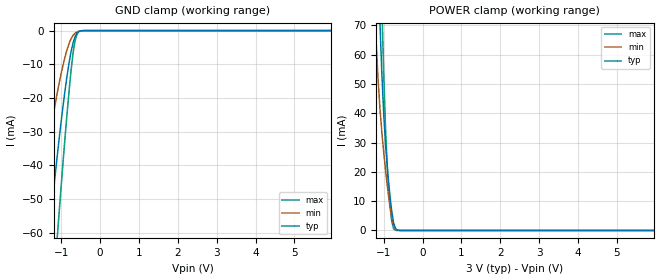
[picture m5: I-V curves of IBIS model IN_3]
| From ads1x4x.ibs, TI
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|   INPUT 3.0V model
[Model]   IN_3
Model_type   Input
| Signals   nRESET, START, nCS, DIN, SCLK
Vinl =  0.45V
Vinh =  1.20V
| variable   typ   min   max
C_comp   7.378pF   8.284pF   6.578pF
[Temperature Range]   40.0   105.0   -40.0
[Voltage range]   5.0V   4.75V   5.25V
[power clamp reference] 3.0V   2.7V   3.3V
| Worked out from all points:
|   GND clamp passes 1 mA (typ) near -0.61 V on its own axis
|   POWER clamp passes 1 mA (typ) near -0.71 V on its own axis
[GND Clamp]
|   Voltage   I(typ)   I(min)   I(max)
-3V       -286.7mA   -194mA     -373.5mA
-1.65V    -102.4mA   -59.28mA   -150mA
-1.3V     -59.09mA   -31.55mA   -92.59mA
-1.1V     -36.8mA    -18.29mA   -60.87mA
-1.05V    -31.64mA   -15.34mA   -53.2mA
-900mV    -17.48mA   -7.66mA    -31.25mA
-750mV    -6.367mA   -2.478mA   -12.03mA
-700mV    -3.772mA   -1.484mA   -6.955mA
-650mV    -1.918mA   -829.5uA   -3.262mA
-600mV    -803.4uA   -434.9uA   -1.177mA
-400mV    -5.931uA   -9.899uA   -2.579uA
5.95V     0A         0A         0A
[POWER Clamp]
|   Voltage   I(typ)   I(min)   I(max)
-3V       1.061A     858mA      1.359A
-1.25V    136.5mA    80.6mA     194.5mA
-1.2V     113.4mA    65.19mA    163.6mA
-1.1V     71.21mA    41.78mA    104.4mA
-1.05V    53.46mA    33.45mA    77mA
-1V       39.14mA    26.36mA    52.5mA
-950mV    28.36mA    19.98mA    32.82mA
-900mV    19.98mA    14.14mA    19.24mA
-850mV    12.96mA    8.929mA    9.991mA
-800mV    7.072mA    4.678mA    3.559mA
-700mV    700.2uA    550.5uA    59.14uA
5.95V     0A         0A         0A
